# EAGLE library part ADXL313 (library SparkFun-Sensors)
Analog Devices ADXL313 3-Axis SPI/I2C 0.5/1/2/4g Ultra Low Power Accelerometer The ADXL313 is a small, thin, low power, 3-axis accelerometer with high resolution (13-bit) measurement up to ±4 g. Digital output data is formatted as 16-bit twos complement and is accessible through either a serial port interface (SPI) (3-wire or 4-wire) or I2C digital interface. Datasheet SparkFun Products SparkFun Triple Axis Accelerometer Breakout - ADXL313 (QWIIC) (SEN-17241)
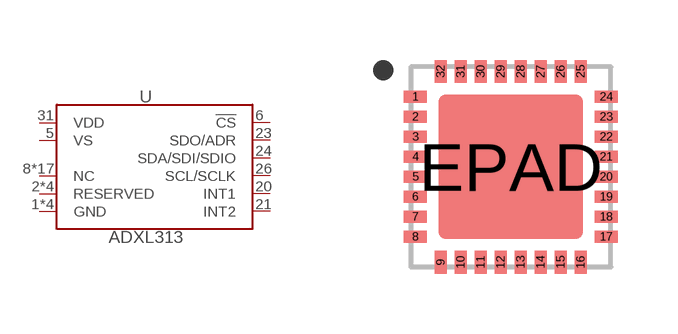
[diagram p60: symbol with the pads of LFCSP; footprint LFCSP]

Designator prefix U

## ADXL313 (PROD_ID: IC-15318)  [LFCSP]
1  GND
2  RESERVED  nc
3  GND
4  GND
5  VS
6  !CS
7  RESERVED  nc
8  NC  nc
9  NC  nc
10  NC  nc
11  NC  nc
12  NC  nc
13  NC  nc
14  NC  nc
15  NC  nc
16  NC  nc
17  NC  nc
18  NC  nc
19  NC  nc
20  INT1
21  INT2
22  RESERVED  nc
23  SDO/ADR
24  SDA/SDI/SDIO
25  NC  nc
26  SCL/SCLK
27  NC  nc
28  NC  nc
29  NC  nc
30  NC  nc
31  VDD
32  RESERVED  nc
EPAD  GND

## Footprint LFCSP (pad centres in mm)
Small and thin: 5 mm × 5 mm × 1.45 mm LFCSP package ADXL313 Datasheet Specifications: Pin Count: 32 Area: 5 x 5 x 1.45 mm Pitch: 0.5 mm Devices Using: ADXL313
smd 0.57 x 0.3: 1 -2.385,1.75; 2 -2.385,1.25; 3 -2.385,0.75; 4 -2.385,0.25; 5 -2.385,-0.25; 6 -2.385,-0.75; 7 -2.385,-1.25; 8 -2.385,-1.75; 17 2.385,-1.75; 18 2.385,-1.25; 19 2.385,-0.75; 20 2.385,-0.25; 21 2.385,0.25; 22 2.385,0.75; 23 2.385,1.25; 24 2.385,1.75
smd 0.3 x 0.57: 9 -1.75,-2.385; 10 -1.25,-2.385; 11 -0.75,-2.385; 12 -0.25,-2.385; 13 0.25,-2.385; 14 0.75,-2.385; 15 1.25,-2.385; 16 1.75,-2.385; 25 1.75,2.385; 26 1.25,2.385; 27 0.75,2.385; 28 0.25,2.385; 29 -0.25,2.385; 30 -0.75,2.385; 31 -1.25,2.385; 32 -1.75,2.385
smd 3.6 x 3.6: EPAD 0,0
